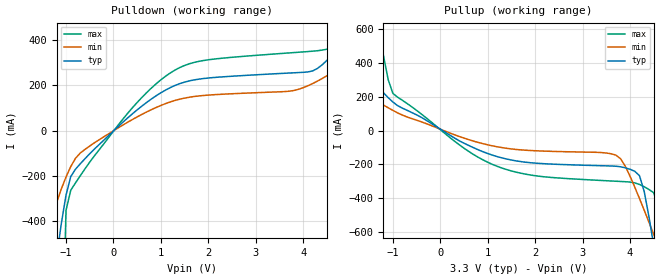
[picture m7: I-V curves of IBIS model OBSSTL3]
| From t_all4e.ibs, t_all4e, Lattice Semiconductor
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|   OBSSTL3
[Model]   OBSSTL3
Model_type   Output
Polarity   Non-Inverting
C_comp   2pF   2pF   2pF
[Temperature Range]   25.0000   125.0000   -40.0000
[Voltage Range]   3.3000V   3.0000V   3.6000V
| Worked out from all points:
|   slope of the pulldown table from 0 to 0.495 V, typ, clamps not added: 5.38 ohm
|   slope of the pullup table from 0 to 0.495 V, typ, clamps not added: 6.01 ohm
[Pulldown]
|voltage   I(typ)   I(min)   I(max)
-3.3V     -4.5A      -1.848A    -40.63A
-1.4V     -905.1mA   -452.3mA   -5.993A
-1.1V     -410.9mA   -257.3mA   -1.16A
-900mV    -202.3mA   -158.6mA   -262.6mA
-800mV    -170.1mA   -122.2mA   -230.3mA
500mV     90.86mA    59.92mA    123.3mA
1.4V      206.4mA    138mA      277.1mA
3.9V      255mA      181.1mA    344.3mA
4.4V      288.9mA    228.6mA    353.8mA
5.1V      460mA      332.3mA    1.049A
5.8V      678.9mA    464.8mA    2.257A
6.6V      955.4mA    633mA      3.701A
[Pullup]
|voltage   I(typ)   I(min)   I(max)
-3.3V     927.1mA    566.9mA    4.204A
-2.4V     605mA      373mA      2.543A
-1.3V     253.8mA    166.6mA    606.4mA
-1.1V     194.3mA    134.5mA    300.9mA
-1V       168.2mA    118.9mA    218.9mA
1.1V      -145.4mA   -90.53mA   -200mA
3.7V      -210.6mA   -144.8mA   -299.2mA
3.9V      -220.1mA   -211.1mA   -302.1mA
4.2V      -266.8mA   -401.8mA   -318.4mA
4.5V      -679.1mA   -613.2mA   -367.7mA
4.7V      -1.036A    -757.5mA   -1.292A
6.6V      -4.632A    -2.166A    -35.28A
[Ramp]
| variable   typ   min   max
dV/dt_r   1.7270/0.2838ns   1.4530/0.5872ns   1.9713/0.1396ns
dV/dt_f   1.7625/0.5630ns   1.5176/1.2649ns   1.9807/0.2594ns
